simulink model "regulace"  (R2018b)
settings: Solver=ode5  StartTime=0.0  StopTime=80  FixedStep=0.01  RelTol=1e-3  AbsTol=1e-6
undefined symbols (not defined in the file or in its folder): Crane3D_Center, Crane3D_RangeBit, Crane3D_ScaleCoeff, rtdac4pciebaseaddress
libraries: simulink x5

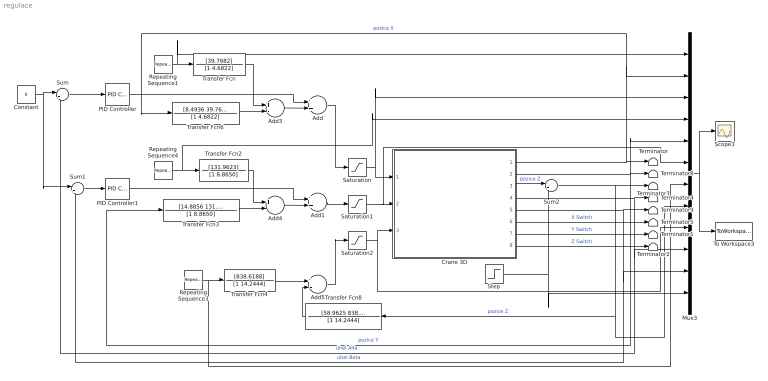
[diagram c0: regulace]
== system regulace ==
  Add : Sum
  Add1 : Sum
  Add3 : Sum  Inputs=+-
  Add4 : Sum  Inputs=+-
  Add5 : Sum  Inputs=+-
  Constant : Constant  Value=0
  Crane 3D : Subsystem  mask{BaseAddress=rtdac4pciebaseaddress, T0=0.01}
      mask prompts: BaseAddress "Base Address:"; T0 "Sampling Period:"
  Mux3 : Mux  Inputs=12
  PID Controller : simulink/Continuous/PID Controller  Controller=P  Form=Parallel  TimeDomain=Continuous-time  SampleTime=-1  IntegratorMethod=Forward Euler  FilterMethod=Forward Euler  ControllerParametersSource=internal  P=-4.5  I=1  D=0  UseFilter=on  N=100  TunerSelectOption=Transfer Function Based (PID Tuner App)  InitialConditionSource=internal  InitialConditionForIntegrator=0  InitialConditionForFilter=0  DifferentiatorICPrevScaledInput=0  ExternalReset=none  TrackingMode=off  Kt=1  LimitOutput=off  UpperSaturationLimit=inf  LowerSaturationLimit=-inf  LinearizeAsGain=on  AntiWindupMode=none  Kb=1  POutMin=[]  POutMax=[]  IOutMin=[]  IOutMax=[]  DOutMin=[]  DOutMax=[]  NOutMin=[]  NOutMax=[]  SumOutMin=[]  SumOutMax=[]  SaturationOutMin=[]  SaturationOutMax=[]  PParamMin=[]  PParamMax=[]  IParamMin=[]  IParamMax=[]  DParamMin=[]  DParamMax=[]  NParamMin=[]  NParamMax=[]  KbParamMin=[]  KbParamMax=[]  KtParamMin=[]  KtParamMax=[]  KbOutMin=[]  KbOutMax=[]  KtOutMin=[]  KtOutMax=[]  IntegratorOutMin=[]  IntegratorOutMax=[]  FilterOutMin=[]  FilterOutMax=[]  SumI1OutMin=[]  SumI1OutMax=[]  SumI2OutMin=[]  SumI2OutMax=[]  SumI3OutMin=[]  SumI3OutMax=[]  SumI4OutMin=[]  SumI4OutMax=[]  SumDOutMin=[]  SumDOutMax=[]  DifferentiatorOutMin=[]  DifferentiatorOutMax=[]  FilterDiffOutCoefMin=[]  FilterDiffOutCoefMax=[]  ReciprocalOutMin=[]  ReciprocalOutMax=[]  SumDenOutMin=[]  SumDenOutMax=[]  SumNumOutMin=[]  SumNumOutMax=[]  DivideOutMin=[]  DivideOutMax=[]  IntegratorContinuousStateAttributes=''  IntegratorStateMustResolveToSignalObject=off  IntegratorRTWStateStorageClass=Auto  FilterContinuousStateAttributes=''  FilterStateMustResolveToSignalObject=off  FilterRTWStateStorageClass=Auto  ParallelPVariant=InternalParameters  IdealPVariant=Disabled  IVariant=Disabled  DVariant=Disabled  IntegratorVariant=Disabled  SatVariant=Disabled  AWVariant=Disabled  PCopyVariant=Disabled  TRVariant=Disabled  FdbkBlocksVariant=Forward  IdealPFdbkVariant=Disabled  SatFdbkVariant=Disabled  DerivativeFilterVariant=Disabled  NVariant=Disabled  NCopyVariant=Disabled_SignalSpec  FilterICVariant=Disabled  IntegratorICVariant=Disabled  ExternalResetVariant=Disabled  TRSumVariant=Passthrough  SumFdbkVariant=Disabled  SumVariant=Passthrough_P
  PID Controller1 : simulink/Continuous/PID Controller  Controller=P  Form=Parallel  TimeDomain=Continuous-time  SampleTime=-1  IntegratorMethod=Forward Euler  FilterMethod=Forward Euler  ControllerParametersSource=internal  P=-4.5  I=1  D=0  UseFilter=on  N=100  TunerSelectOption=Transfer Function Based (PID Tuner App)  InitialConditionSource=internal  InitialConditionForIntegrator=0  InitialConditionForFilter=0  DifferentiatorICPrevScaledInput=0  ExternalReset=none  TrackingMode=off  Kt=1  LimitOutput=off  UpperSaturationLimit=inf  LowerSaturationLimit=-inf  LinearizeAsGain=on  AntiWindupMode=none  Kb=1  POutMin=[]  POutMax=[]  IOutMin=[]  IOutMax=[]  DOutMin=[]  DOutMax=[]  NOutMin=[]  NOutMax=[]  SumOutMin=[]  SumOutMax=[]  SaturationOutMin=[]  SaturationOutMax=[]  PParamMin=[]  PParamMax=[]  IParamMin=[]  IParamMax=[]  DParamMin=[]  DParamMax=[]  NParamMin=[]  NParamMax=[]  KbParamMin=[]  KbParamMax=[]  KtParamMin=[]  KtParamMax=[]  KbOutMin=[]  KbOutMax=[]  KtOutMin=[]  KtOutMax=[]  IntegratorOutMin=[]  IntegratorOutMax=[]  FilterOutMin=[]  FilterOutMax=[]  SumI1OutMin=[]  SumI1OutMax=[]  SumI2OutMin=[]  SumI2OutMax=[]  SumI3OutMin=[]  SumI3OutMax=[]  SumI4OutMin=[]  SumI4OutMax=[]  SumDOutMin=[]  SumDOutMax=[]  DifferentiatorOutMin=[]  DifferentiatorOutMax=[]  FilterDiffOutCoefMin=[]  FilterDiffOutCoefMax=[]  ReciprocalOutMin=[]  ReciprocalOutMax=[]  SumDenOutMin=[]  SumDenOutMax=[]  SumNumOutMin=[]  SumNumOutMax=[]  DivideOutMin=[]  DivideOutMax=[]  IntegratorContinuousStateAttributes=''  IntegratorStateMustResolveToSignalObject=off  IntegratorRTWStateStorageClass=Auto  FilterContinuousStateAttributes=''  FilterStateMustResolveToSignalObject=off  FilterRTWStateStorageClass=Auto  ParallelPVariant=InternalParameters  IdealPVariant=Disabled  IVariant=Disabled  DVariant=Disabled  IntegratorVariant=Disabled  SatVariant=Disabled  AWVariant=Disabled  PCopyVariant=Disabled  TRVariant=Disabled  FdbkBlocksVariant=Forward  IdealPFdbkVariant=Disabled  SatFdbkVariant=Disabled  DerivativeFilterVariant=Disabled  NVariant=Disabled  NCopyVariant=Disabled_SignalSpec  FilterICVariant=Disabled  IntegratorICVariant=Disabled  ExternalResetVariant=Disabled  TRSumVariant=Passthrough  SumFdbkVariant=Disabled  SumVariant=Passthrough_P
  Repeating Sequence1 : simulink/Sources/Repeating Sequence  rep_seq_t=[0 14.99 15 24.99 25 39.99 40 54.99 55 64.99 65 80]  rep_seq_y=[0.001 0.001 0.4 0.4 0.1 0.1 0.3 0.3 0.5 0.5 Crane3D_Center('X') Crane3D_Center('X')]
  Repeating Sequence3 : simulink/Sources/Repeating Sequence  rep_seq_t=[0 4.99 5 19.99 20 34.99 35 49.99 50 64.99 65 80]  rep_seq_y=[0.001 0.001 0.1 0.1 0.2 0.2 0.3 0.3 0.4 0.4 0.5 0.5]
  Repeating Sequence4 : simulink/Sources/Repeating Sequence  rep_seq_t=[0 7.99 8 29.99 30 39.99 40 59.99 60 69.99 70 80]  rep_seq_y=[0.2 0.2 0.1 0.1 0.5 0.5 0.3 0.3 0.4 0.4 Crane3D_Center('Y') Crane3D_Center('Y')]
  Saturation : Saturate  UpperLimit=1  LowerLimit=-1
  Saturation1 : Saturate  UpperLimit=1  LowerLimit=-1
  Saturation2 : Saturate  UpperLimit=1  LowerLimit=-1
  Scope3 : Scope
  Step : Step  Time=12  After=0.1  SampleTime=0
  Sum : Sum  Inputs=|+-
  Sum1 : Sum  Inputs=|+-
  Sum2 : Sum  Inputs=|++
  Terminator{,1..5,8..9} (8 alike) : Terminator
  To Workspace3 : ToWorkspace  VariableName=CraneReg  SaveFormat=Timeseries  SampleTime=-1
  Transfer Fcn : TransferFcn  Numerator=[39.7682]  Denominator=[1 4.6822]
  Transfer Fcn2 : TransferFcn  Numerator=[131.9623]  Denominator=[1 8.8650]
  Transfer Fcn3 : TransferFcn  Numerator=[14.8856 131.9623]  Denominator=[1 8.8650]
  Transfer Fcn4 : TransferFcn  Numerator=[838.6188]  Denominator=[1 14.2444]
  Transfer Fcn6 : TransferFcn  Numerator=[8.4936 39.7682]  Denominator=[1 4.6822]
  Transfer Fcn8 : TransferFcn  Numerator=[58.9625 838.6188]  Denominator=[1 14.2444]
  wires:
  Transfer Fcn4/1 -> Add5/1
  Add/1 -> Saturation/1
  Sum1/1 -> PID Controller1/1
  Add4/1 -> Add1/2
  Transfer Fcn3/1 -> Add4/2
  Add1/1 -> Saturation1/1
  Transfer Fcn2/1 -> Add4/1
  Repeating Sequence3/1 -> Mux3/7, Transfer Fcn4/1
  Sum2/1 -> Mux3/8, Transfer Fcn8/1, Terminator3/1  "pozice Z"
  Transfer Fcn8/1 -> Add5/2
  Constant/1 -> Sum1/1, Sum/1
  Transfer Fcn6/1 -> Add3/2
  Sum/1 -> PID Controller/1
  PID Controller/1 -> Add/1
  Add5/1 -> Saturation2/1
  Repeating Sequence1/1 -> Mux3/1, Transfer Fcn/1
  Add3/1 -> Add/2
  Mux3/1 -> To Workspace3/1, Scope3/1
  Transfer Fcn/1 -> Add3/1
  Crane 3D/1(X Position) -> Mux3/2, Transfer Fcn6/1, Terminator/1  "pozice X"
  Crane 3D/3(Z Position) -> Sum2/1  "pozice Z"
  Step/1 -> Mux3/12, Sum2/2
  Repeating Sequence4/1 -> Mux3/4, Transfer Fcn2/1
  Crane 3D/2(Y Position) -> Transfer Fcn3/1, Mux3/5, Terminator8/1  "pozice Y"
  Crane 3D/7(Y Switch) -> Terminator1/1  "Y Switch"
  Crane 3D/6(X Switch) -> Terminator5/1  "X Switch"
  Crane 3D/5(Y Angle) -> Terminator9/1, Sum1/2, Mux3/11  "úhel Beta"
  Crane 3D/4(X Angle) -> Terminator4/1, Mux3/10, Sum/2  "úhel Alfa"
  Crane 3D/8(Z Switch) -> Terminator2/1  "Z Switch"
  PID Controller1/1 -> Add1/1
  Saturation/1 -> Mux3/3, Crane 3D/1(X PWM)
  Saturation1/1 -> Mux3/6, Crane 3D/2(Y PWM)
  Saturation2/1 -> Mux3/9, Crane 3D/3(Z PWM)

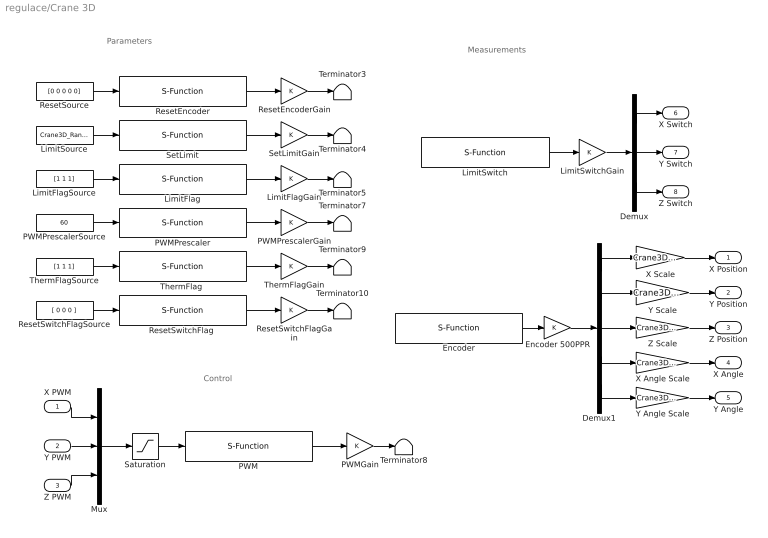
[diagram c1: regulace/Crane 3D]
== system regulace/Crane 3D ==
  note: Parameters
  note: Control
  note: Measurements
  X PWM : Inport
  Y PWM : Inport  Port=2
  Z PWM : Inport  Port=3
  Demux : Demux  Outputs=3
  Demux1 : Demux  Outputs=5
  Encoder : S-Function  FunctionName=Crane3D_Encoder  Parameters=BaseAddress, T0  SFunctionDeploymentMode=off  EnableBusSupport=off
  Encoder 500PPR : Gain
  LimitFlag : S-Function  FunctionName=Crane3D_LimitFlag  Parameters=BaseAddress, T0  SFunctionDeploymentMode=off  EnableBusSupport=off
  LimitFlagGain : Gain
  LimitFlagSource : Constant  Value=[1 1 1]
  LimitSource : Constant  Value=Crane3D_RangeBit
  LimitSwitch : S-Function  FunctionName=Crane3D_Switch  Parameters=BaseAddress, T0  SFunctionDeploymentMode=off  EnableBusSupport=off
  LimitSwitchGain : Gain
  Mux : Mux  Inputs=3
  PWM : S-Function  FunctionName=Crane3D_PWM  Parameters=BaseAddress, T0  SFunctionDeploymentMode=off  EnableBusSupport=off
  PWMGain : Gain
  PWMPrescaler : S-Function  FunctionName=Crane3D_PWMPrescaler  Parameters=BaseAddress, T0  SFunctionDeploymentMode=off  EnableBusSupport=off
  PWMPrescalerGain : Gain
  PWMPrescalerSource : Constant  Value=60
  ResetEncoder : S-Function  FunctionName=Crane3D_ResetEncoder  Parameters=BaseAddress, T0  SFunctionDeploymentMode=off  EnableBusSupport=off
  ResetEncoderGain : Gain
  ResetSource : Constant  Value=[0 0 0 0 0]
  "ResetSwitchFlag " : S-Function  FunctionName=Crane3D_ResetSwitchFlag  Parameters=BaseAddress, T0  SFunctionDeploymentMode=off  EnableBusSupport=off
  ResetSwitchFlagGain : Gain
  ResetSwitchFlagSource : Constant  Value=[ 0 0 0 ]
  Saturation : Saturate  UpperLimit=1  LowerLimit=-1
  SetLimit : S-Function  FunctionName=Crane3D_SetLimit  Parameters=BaseAddress, T0  SFunctionDeploymentMode=off  EnableBusSupport=off
  SetLimitGain : Gain
  Terminator{3..5,7..10} (7 alike) : Terminator
  "ThermFlag " : S-Function  FunctionName=Crane3D_ThermFlag  Parameters=BaseAddress, T0  SFunctionDeploymentMode=off  EnableBusSupport=off
  ThermFlagGain : Gain
  ThermFlagSource : Constant  Value=[1 1 1]
  X Angle Scale : Gain  Gain=Crane3D_ScaleCoeff( 4 )
  X Scale : Gain  Gain=Crane3D_ScaleCoeff( 1 )
  Y Angle Scale : Gain  Gain=Crane3D_ScaleCoeff( 5 )
  Y Scale : Gain  Gain=Crane3D_ScaleCoeff( 2 )
  Z Scale : Gain  Gain=Crane3D_ScaleCoeff( 3 )
  X Position : Outport  InitialOutput=0
  Y Position : Outport  Port=2  InitialOutput=0
  Z Position : Outport  Port=3  InitialOutput=0
  X Angle : Outport  Port=4  InitialOutput=0
  Y Angle : Outport  Port=5  InitialOutput=0
  X Switch : Outport  Port=6  InitialOutput=0
  Y Switch : Outport  Port=7  InitialOutput=0
  Z Switch : Outport  Port=8  InitialOutput=0
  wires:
  Encoder 500PPR/1 -> Demux1/1
  Encoder/1 -> Encoder 500PPR/1
  Saturation/1 -> PWM/1
  Mux/1 -> Saturation/1
  PWM/1 -> PWMGain/1
  PWMGain/1 -> Terminator8/1
  ResetEncoder/1 -> ResetEncoderGain/1
  SetLimit/1 -> SetLimitGain/1
  LimitFlag/1 -> LimitFlagGain/1
  PWMPrescaler/1 -> PWMPrescalerGain/1
  "ThermFlag "/1 -> ThermFlagGain/1
  "ResetSwitchFlag "/1 -> ResetSwitchFlagGain/1
  ResetSource/1 -> ResetEncoder/1
  LimitSource/1 -> SetLimit/1
  LimitFlagSource/1 -> LimitFlag/1
  PWMPrescalerSource/1 -> PWMPrescaler/1
  ThermFlagSource/1 -> "ThermFlag "/1
  ResetSwitchFlagSource/1 -> "ResetSwitchFlag "/1
  ResetEncoderGain/1 -> Terminator3/1
  SetLimitGain/1 -> Terminator4/1
  LimitFlagGain/1 -> Terminator5/1
  PWMPrescalerGain/1 -> Terminator7/1
  ThermFlagGain/1 -> Terminator9/1
  ResetSwitchFlagGain/1 -> Terminator10/1
  Z PWM/1 -> Mux/3
  Y PWM/1 -> Mux/2
  X PWM/1 -> Mux/1
  LimitSwitch/1 -> LimitSwitchGain/1
  LimitSwitchGain/1 -> Demux/1
  Demux/1 -> X Switch/1
  Demux/2 -> Y Switch/1
  Demux/3 -> Z Switch/1
  Z Scale/1 -> Z Position/1
  X Scale/1 -> X Position/1
  Y Scale/1 -> Y Position/1
  Y Angle Scale/1 -> Y Angle/1
  X Angle Scale/1 -> X Angle/1
  Demux1/5 -> Y Angle Scale/1
  Demux1/4 -> X Angle Scale/1
  Demux1/3 -> Z Scale/1
  Demux1/2 -> Y Scale/1
  Demux1/1 -> X Scale/1
